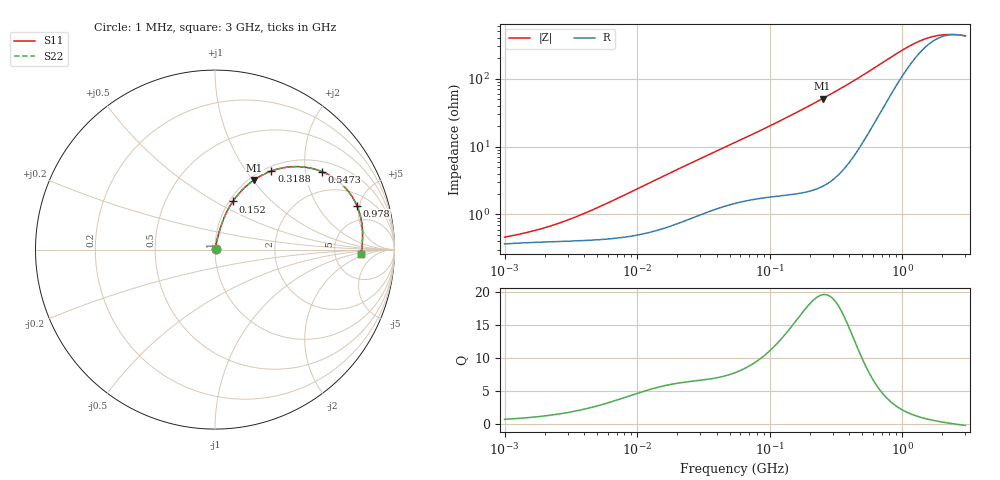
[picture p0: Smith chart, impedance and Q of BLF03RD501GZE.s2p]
! BLF03RD501GZE
# Hz S RI R 50
!Freq.(Hz) S11(Real) S11(Imag) S21(Real) S21(Imag) S12(Real) S12(Imag) S22(Real) S22(Imag)
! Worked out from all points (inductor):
!   401 points, 1 MHz to 3 GHz, reference 50 ohm
!   read as one part in series: L = 37.4 nH near 5.481 MHz
!   highest Q = 19.6 at 250.7 MHz (marker M1), where L = 32.3 nH
!   self-resonance near 2.602 GHz
!   S11 on the Smith chart (normalised r, x): 1 MHz: 1.01, +0.01; 152 MHz: 1.04, +0.61; 318.8 MHz: 1.07, +1.32; 547.3 MHz: 1.30, +2.48; 978 MHz: 3.04, +4.72; 3 GHz: 9.51, -1.44
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1000000  0.00368 0.00279  0.9963 -0.00279  0.9963 -0.00279  0.00368 0.00279
1974946  0.00394 0.00491  0.9961 -0.00491  0.9961 -0.00491  0.00394 0.00491
2720446  0.00404 0.00656  0.996 -0.00656  0.996 -0.00656  0.00404 0.00656
3823119  0.00418 0.00905  0.9958 -0.00905  0.9958 -0.00905  0.00418 0.00905
6305767  0.00459 0.0147  0.9954 -0.0147  0.9954 -0.0147  0.00459 0.0147
1.461624e7  0.00701 0.0332  0.993 -0.0332  0.993 -0.0332  0.00701 0.0332
3.00453e7  0.014 0.0645  0.986 -0.0645  0.986 -0.0645  0.014 0.0645
5.477226e7  0.0267 0.1094  0.9733 -0.1094  0.9733 -0.1094  0.0267 0.1094
9.216659e7  0.049 0.1734  0.951 -0.1734  0.951 -0.1734  0.049 0.1734
1.520175e8  0.0993 0.268  0.9007 -0.268  0.9007 -0.268  0.0993 0.268
2.094008e8  0.164 0.3444  0.836 -0.3444  0.836 -0.3444  0.164 0.3444
2.507343e8  0.2182 0.3883  0.7818 -0.3883  0.7818 -0.3883  0.2182 0.3883
3.188066e8  0.3145 0.438  0.6855 -0.438  0.6855 -0.438  0.3145 0.438
4.219165e8  0.4575 0.4623  0.5425 -0.4623  0.5425 -0.4623  0.4575 0.4623
5.473095e8  0.5977 0.4337  0.4023 -0.4337  0.4023 -0.4337  0.5977 0.4337
6.685918e8  0.6888 0.3793  0.3112 -0.3793  0.3112 -0.3793  0.6888 0.3793
8.005644e8  0.7489 0.3167  0.2511 -0.3167  0.2511 -0.3167  0.7489 0.3167
9.779672e8  0.7906 0.2445  0.2094 -0.2445  0.2094 -0.2445  0.7906 0.2445
1.347129e9  0.8183 0.1437  0.1817 -0.1437  0.1817 -0.1437  0.8183 0.1437
1.747494e9  0.8224 0.0791  0.1776 -0.0791  0.1776 -0.0791  0.8224 0.0791
2.266846e9  0.8198 0.0256  0.1802 -0.0256  0.1802 -0.0256  0.8198 0.0256
3e9  0.8133 -0.0256  0.1867 0.0256  0.1867 0.0256  0.8133 -0.0256
